DATA_BLOCK     DRIVDB90
TITLE=         DRIVDB90
AUTHOR:        DRVDPS7
FAMILY:        DRIVES
NAME:          DRIVDB90
VERSION:       5.5

STRUCT
   SLAVE_3                     : STRUCT
       DPADDR                  : WORD;           // PROFIBUS address / device number of the slave
       DADDR                   : WORD;           // Diagnostics address of the slave
       SLOT_4                  : SLOT_UDT;       // Slot-specific configuration data Slot 4
       SLOT_5                  : SLOT_UDT;       // Slot-specific configuration data Slot 5
       SLOT_7                  : SLOT_UDT;       // Slot-specific configuration data Slot 7
       SLOT_8                  : SLOT_UDT;       // Slot-specific configuration data Slot 8
   END_STRUCT;

END_STRUCT;


BEGIN
   // SLAVE_3
   SLAVE_3.DPADDR              := W#16#3;        // PROFIBUS address / device number of the slave: 3
   SLAVE_3.DADDR               := W#16#3FE;      // Diagnostics address of the slave: 1022
   SLAVE_3.SLOT_4.LADDR        := W#16#110;      // I/O base address of the slot: 272
   SLAVE_3.SLOT_4.SLOT_ID      := B#16#2;        // Slot type designation: 2
   SLAVE_3.SLOT_4.PCD_ADDR     := B#16#1;        // Process data start address for setpoint and/or actual value slot: 1
   SLAVE_3.SLOT_4.LENGTH       := B#16#6;        // Length in words of slot data to be transferred: 6
   SLAVE_3.SLOT_4.CONSIST      := TRUE;          // Consistency: Total length
   SLAVE_3.SLOT_5.LADDR        := W#16#110;      // I/O base address of the slot: 272
   SLAVE_3.SLOT_5.SLOT_ID      := B#16#1;        // Slot type designation: 1
   SLAVE_3.SLOT_5.PCD_ADDR     := B#16#1;        // Process data start address for setpoint and/or actual value slot: 1
   SLAVE_3.SLOT_5.LENGTH       := B#16#6;        // Length in words of slot data to be transferred: 6
   SLAVE_3.SLOT_5.CONSIST      := TRUE;          // Consistency: Total length
   SLAVE_3.SLOT_7.LADDR        := W#16#11C;      // I/O base address of the slot: 284
   SLAVE_3.SLOT_7.SLOT_ID      := B#16#2;        // Slot type designation: 2
   SLAVE_3.SLOT_7.PCD_ADDR     := B#16#1;        // Process data start address for setpoint and/or actual value slot: 1
   SLAVE_3.SLOT_7.LENGTH       := B#16#2;        // Length in words of slot data to be transferred: 2
   SLAVE_3.SLOT_7.CONSIST      := FALSE;         // Consistency: Unit
   SLAVE_3.SLOT_8.LADDR        := W#16#11C;      // I/O base address of the slot: 284
   SLAVE_3.SLOT_8.SLOT_ID      := B#16#1;        // Slot type designation: 1
   SLAVE_3.SLOT_8.PCD_ADDR     := B#16#1;        // Process data start address for setpoint and/or actual value slot: 1
   SLAVE_3.SLOT_8.LENGTH       := B#16#2;        // Length in words of slot data to be transferred: 2
   SLAVE_3.SLOT_8.CONSIST      := FALSE;         // Consistency: Unit

END_DATA_BLOCK
